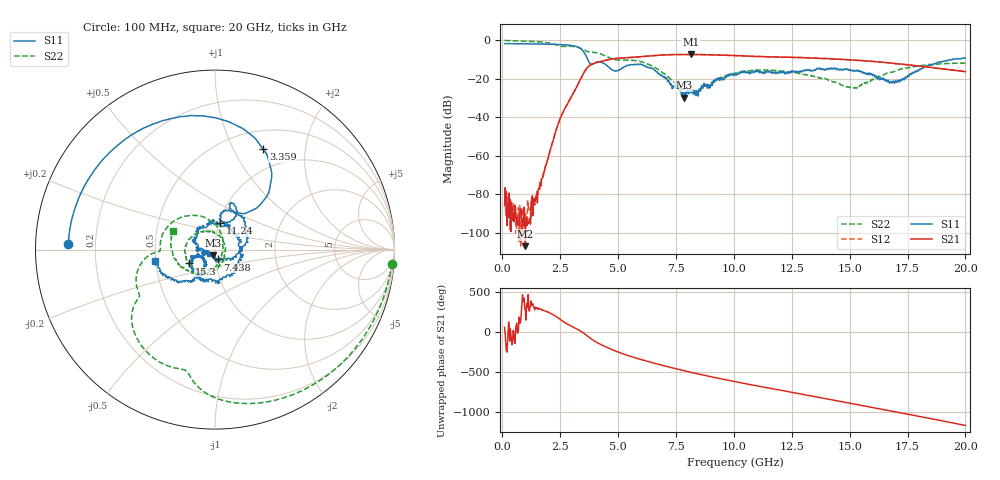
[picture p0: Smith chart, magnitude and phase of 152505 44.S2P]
!  2-Port S-parameters saved by WinCal
! VAR MeasName=S-Parameters (CALIBRATED_DATA) read from VNA (N5230C)
! VAR MeasDate=4/10/2015 9:32:52 AM
! VAR NAME=152505 44
! VAR FILENAME=152505 44.S2P
! VAR DATE=4/10/2015 9:32:52 AM
! VAR PHYS_PORTS=1,2
# Hz S DB R 50
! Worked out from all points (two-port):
!   801 points, 100 MHz to 20 GHz, reference 50 ohm
!   highest |S21| = -7.37 dB at 8.135 GHz (marker M1); lowest = -107.1 dB at 995.5 MHz (marker M2)
!   |S21| within 3 dB of the highest: 4.456 GHz to 15.28 GHz (10.83 GHz wide, 110 % of centre)
!   lowest |S11| = -29.8 dB at 7.836 GHz (marker M3), VSWR 1.07, Z = 48.8 - j2.97 ohm
!   |S11| at or under -10 dB: 3.694 GHz to 19.43 GHz (15.74 GHz wide, 136 % of centre)
!   |S22| runs from -27.3 to -0.1 dB; largest |S21 - S12| = 0.0058
!   S11 on the Smith chart (normalised r, x): 100 MHz: 0.10, +0.02; 3.359 GHz: 0.73, +1.32; 7.438 GHz: 1.03, -0.11; 11.24 GHz: 1.01, +0.30; 15.3 GHz: 0.74, -0.12; 20 GHz: 0.49, -0.07
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1e8  -1.75 177.7  -86.12 55.8  -80.57 81.8  -0.08 -4.6
9.955e8  -1.83 156.1  -107.09 -93.9  -90.21 70.7  -0.45 -40.3
1.567625e9  -1.92 141.4  -77.04 -78.0  -77.67 -60.3  -0.80 -64.0
2.463125e9  -2.20 113.4  -41.88 161.6  -41.86 161.4  -2.92 -101.5
3.358625e9  -4.14 64.3  -20.66 11.4  -20.67 11.9  -4.02 -136.8
3.43325e9  -4.85 58.2  -18.88 -2.1  -18.89 -1.8  -4.39 -140.4
3.905875e9  -12.37 67.2  -12.19 -102.7  -12.21 -102.5  -6.26 -151.4
4.453125e9  -12.52 60.3  -10.38 173.0  -10.42 173.0  -8.13 -172.7
5.249125e9  -13.90 80.1  -9.14 79.5  -9.14 79.7  -10.32 176.6
6.02025e9  -12.80 46.0  -8.52 10.9  -8.51 10.9  -11.24 142.9
6.741625e9  -17.50 -4.1  -7.78 -46.2  -7.78 -46.4  -15.30 102.4
7.438125e9  -24.89 -74.0  -7.43 -97.8  -7.42 -97.8  -22.00 60.0
7.836125e9  -29.80 -110.0  -7.40 -125.7  -7.38 -125.5  -26.45 25.5
8.134625e9  -27.21 -136.0  -7.37 -145.5  -7.39 -145.5  -27.09 -4.3
8.980375e9  -24.69 -175.9  -7.54 160.3  -7.54 160.5  -22.58 -75.9
1.005e10  -17.44 150.7  -7.92 97.3  -7.96 97.0  -17.08 -124.5
1.1244e10  -16.49 78.7  -8.46 31.7  -8.48 31.8  -15.50 -169.9
1.338325e10  -15.55 -68.5  -9.21 -83.1  -9.14 -82.8  -18.59 121.8
1.529862e10  -15.74 -151.9  -10.40 173.0  -10.30 172.7  -24.94 -16.4
1.669162e10  -21.35 -146.3  -11.73 96.1  -11.76 95.5  -16.85 -110.9
1.8209e10  -13.85 -126.2  -13.78 12.2  -13.65 12.5  -13.15 -163.4
2e10  -9.29 -168.9  -16.29 -88.7  -16.28 -88.6  -11.86 155.7
